FUNCTION "fc_CP_Send" : VOID
TITLE =Send CP data -PMA systembus-
//version!date    !author !change_segm!change_description
//-------+--------+-------+-----------+-------------------------------
// 1.0   !21.05.00!Kahle  ! ---       ! 1st version
// 1.1   !25.09.00!Kahle  ! 4         ! startOrder =true
//       !        !       ! 5         ! check if own station faulty
// 1.2   !10.11.00!Kahle  ! 6         ! act. tieBrk config instead of the
//       !        !       !           ! compl.config.
// 1.3   !12.03.01!Kahle  ! 6         ! if signal "OUT_uncond_semi" true the
//       !        !       !           ! signal "OUT_moreCPFaulty" is also true
// 1.4   !17.06.01!Kahle  ! 4         ! new para.: mem_actStation
//       !        !       !           ! if status =0 (Call FC5 "AG_Send")
//       !        !       !           ! --> #act_linkCond =true
//       !        !       !           ! No. of sending stations are limited per
//       !        !       !           ! call.
//       !        !       !           ! corr. delete receive buffer in case of
//       !        !       !           ! link failure
//                                                                              !
//Send CP data:
//          For each destination station exist a send data area.
//          Dependent the plant configuration are send the data to the
//          corresponding stations.
//          In case of a failure it be set an indication.
//
AUTHOR : Kahle
FAMILY : PMA71
NAME : SendFDL
VERSION : 1.4


VAR_OUTPUT
  OUT_uncond_semi : BOOL ;	//unconditional semi automatic (semi OP or semi)
  OUT_CPFaulty : BOOL ;	//At least one essential CP stations are faulty
  OUT_moreCPFaulty : BOOL ;	//more than one essential CP stations are faulty
END_VAR
VAR_IN_OUT
  mem_linkCond : DWORD ;	//link condition of each participent (=0:no order/ =1:order running)
  mem_actStation : BYTE ;	//last valid station to that data it was sent
END_VAR
VAR_TEMP
  status : WORD ;	//status value FC5 "AG_SEND"
  done : BOOL ;	//done FC5 "AG_SEND"
  error : BOOL ;	//error flag FC5 "AG_SEND"
  startOrder : BOOL ;	//=1: start order, =0:check running order
  act_linkCond : BOOL ;	//link condition of the actual participent
  no_comm : BOOL ;	//no communication possible
  send_release : BOOL ;	//send release
  newStationSend : BOOL ;	//in the loop the first order
  life_rcv : BOOL ;	//received life signal
  no_actStation : BYTE ;	//Number of stations to which data is sent
  return : INT ;	//return value function "FILL"
  REQ_ID : DWORD ;	//-- not vaild --
  data_pointer : ANY ;	//source area for the received data
  link_cnt : INT ;	//loop counter send link
  participant : DWORD ;	//CP participants (.0:G1 -.14:G15;.15:EG;.16:T1 -.19:T4;.20:S1;.21:S2
  timer_CP : INT ;	//number of the actual monitoring timer 'CP link'
  byte_bit_fail : INT ;	//byte.bit address of the CP link failure of the actual participant
  faulty_stations : DWORD ;	//faulty CP stations
  no_faulty : BYTE ;	//number of faulty CP stations
  ownStation_mask : DWORD ;	//faulty mask own station
  act_link : INT ;	//number of the actual link
  cnt_linkID : BYTE ;	//counter 'determine the link ID'
  link_fail : BOOL ;	//link failure to the actual station
END_VAR
BEGIN
NETWORK
TITLE =inital. internal variables

      CLR   ;
      =     #OUT_uncond_semi;
      =     #newStationSend;
      L     0;
      T     #no_actStation;
NETWORK
TITLE =Send CP data -inital. int.var -
// ANY-pointer: Send MPI data  (P#DB105.DBX0.0 BYTE 30)
      L     B#16#10;
      T     LB    10; //ANY-pointer: 16#10
      L     2;
      T     LB    11; //ANY-pointer: datatyp BYTE
      L     30;
      T     LW    12; //ANY-pointer: repeat factor
      L     105;
      T     LW    14; //ANY-pointer: DB No.
      L     P#DBX 0.0;
      T     LD    16; //ANY-pointer: DBX No.


NETWORK
TITLE =Check of the net configuration

      L     "prm_pma".p_tiebrkCfg;
      L     B#16#F;
      UW    ;
      L     "prm_pma".p_cfg11;
      RLD   4;
      OD    ;
      T     #participant; //actual participants

NETWORK
TITLE =Send CP data - Send data -

//verify whether the last active station is valid
      U(    ;
      L     #mem_actStation;
      L     0;
      >I    ;
      )     ;
      U(    ;
      L     20;
      L     #mem_actStation;
      >=I   ;
      )     ;
      SPB   lpsd; // if mem_actStation vaild -->jump
      L     20; // or mem_actStation not valid -->set =station 20

//Loop send data
lpsd: T     #link_cnt;
      L     #participant;
      SRD   ;
      SPZ   nxt; //participant'x' not defined ...next one

//check if destination =own station
      L     "prm_pma".p_station;
      L     #link_cnt;
      ==I   ;
      SPB   nxt; //if destination address =own station then ..next link

//actual station defined & not the own station
      L     #no_actStation;
      +     1;
      T     #no_actStation;

//source address for send data determined
      L     P#DBX 0.0;
      T     LD    16; //ANY-pointer: DBX No. -Send-
      L     #link_cnt;
      +     104;
      T     LW    14; //ANY-pointer: DB No.

//determine the link failure address
      L     #link_cnt;
      +     -1;
      L     8;
      /I    ;
      SLW   3; //convert byte ->pointer
      PUSH  ;
      RRD   16;
      OW    ;
      L     W#16#FFFF;
      UD    ;
      LAR1  ; //relative byte.bit address of the link failure of the actual participant
      T     #byte_bit_fail;

//Send data - life signal - calculate actual timer
      L     #link_cnt;
      +     100;
      T     #timer_CP; //actual Timer (participant +100)

//Send data - life signal - check the link status of each participant
      AUF   "diagn";
      UN    T [#timer_CP]; //timer stopped -->link failure
      UN    DBX [AR1,P#60.0];
      SPBN  chkT;
      S     DBX [AR1,P#60.0]; //sfc failure of the actual participant
      S     M [AR1,P#120.0]; //if monitoring time run out OR sfc failure then ...link failure
      S     #link_fail;

//link failure -reset receive buffer
      L     0;
      T     MB   255; //presetting for the receive buffer
      L     P#DBX 30.0;
      T     LD    16; //ANY-pointer: DBX No. -Receive-
      CALL "FILL" (
           BVAL                     := P#M 255.0 BYTE 1,
           RET_VAL                  := #return,
           BLK                      := #data_pointer);//the receive buffer is preset with zero

//check link status
chkT: AUF   DB [LW 14];
      U     DBX   31.7; //c_lifeG1
      L     "prm_pma".p_moniTimeMPI;
      SV    T [#timer_CP]; //..start monitoring time of the actual participant
      AUF   DB [LW 14];
      R     DBX   31.7;
      AUF   "diagn";
      R     M [AR1,P#120.0]; //reset link failure
      R     DBX [AR1,P#60.0]; //reset sfc failure of the actual participant
      R     #link_fail;

//send data -faulty order- reset commands
//      AUF   DB [LW 14]
//      L     DBD    0
//      L     DW#16#800000                //c_life
//      UD
//     T     DBD    0

//################################# especially CP Profibus ######################################################
//read the actual link condition
      L     #link_cnt;
      L     #mem_linkCond;
      SRD   ;
      SET   ;
      SPP   lnkC;
      CLR   ;
lnkC: =     #act_linkCond; //link condition of the actual participent =1 : order is finished or not started

//determine the link-ID
      L     0;
      T     #act_link;
      L     20;
lpID: T     #cnt_linkID;
      L     #participant;
      SRD   ;
      SPZ   nxID; //participant'x' not defined ...check the next ID

      L     "prm_pma".p_station;
      L     #cnt_linkID;
      ==I   ;
      SPB   nxID; //destination address =own station ...check next ID

      L     #act_link;
      +     1;
      T     #act_link;

      L     #link_cnt;
      L     #cnt_linkID;
      ==I   ;
      SPB   snd; //counter =act.link ...link ID defined
nxID: L     #cnt_linkID;
      LOOP  lpID;


//send data -check actual order running or start new order-
snd:  U     #act_linkCond;
      =     #startOrder;
//***************************************************************************************************************
      CALL "AG_SEND" (
           ACT                      := #startOrder,
           ID                       := #act_link,
           LADDR                    := "prm_pma".p_CP_add,
           SEND                     := #data_pointer,
           LEN                      := LW    12,//number of byte
           DONE                     := #done,
           ERROR                    := #error,
           STATUS                   := #status);
//***************************************************************************************************************
      L     #status; //if status =0 then ...actual order finished or no order is started
      L     0;
      ==I   ;
      =     #act_linkCond;


//################################# especially CP_Profibus ######################################################

//store the link condition
      L     #link_cnt;
      L     DW#16#80000000; //set bit32
      RLD   ; //bit position of the actual participent
      U     #act_linkCond;
      SPB   sLnk; //if act_linkCond =true then ...set
      INVD  ;
      L     #mem_linkCond;
      UW    ;
      T     #mem_linkCond; //reset link condition
      SPA   nxt;
sLnk: L     #mem_linkCond;
      OW    ;
      T     #mem_linkCond; //set link condition

//maximum numbers of station per call is achieved ?
nxt:  U(    ;
      L     #no_actStation;
      L     0;
      >I    ;
      )     ;
      U(    ;
      L     #no_actStation;
      L     DB41.DBB   40;
      >=I   ;
      )     ;
      SPB   lend; //Number of stations per call to which data are sent is achieved

//at least one defined station are verified ?
      O(    ;
      L     #no_actStation;
      L     0;
      <>I   ;
      )     ;
      O(    ;
      L     #link_cnt;
      L     1;
      <>I   ;
      )     ;
      SPB   nx;
//no defined stations are verified
      L     21;
      T     #link_cnt; //Start the verification at the beginning

//next station
nx:   L     #link_cnt;
      LOOP  lpsd;

//after the end of the loop
lend: L     #link_cnt;
      +     -1;
      T     #mem_actStation; //Storing the station which comes after the station to which data were sent at last
NETWORK
TITLE =Check if own station faulty

      L     "prm_pma".p_tiebrkCfg;
      L     B#16#F;
      UW    ;
      L     "prm_pma".p_cfg11;
      RLD   4;
      OD    ;
      T     #participant; //actual participants

      L     "prm_pma".p_station;
      L     DW#16#80000000;
      RLD   ;
      T     #ownStation_mask; // mask 'own station'

      L     #participant;
      L     #ownStation_mask;
      INVD  ;
      UD    ; //all participants without own station
      L     MD   120;
      TAD   ;
      <>D   ;
      O(    ;
      L     0;
      ==D   ;
      )     ; //if no all foreign stations faulty then ...reset own station
      SPB   Rown; //  or no faulty stations

// all stations faulty
      L     #ownStation_mask;
      TAD   ;
      L     MD   120;
      OD    ;
      T     MD   120; //set own station as faulty
      SPA   unSe;
// not all stations faulty
Rown: L     #ownStation_mask;
      INVD  ;
      TAD   ;
      L     MD   120;
      UD    ;
      T     MD   120; //set own station as o.k.

NETWORK
TITLE =Check if CP failure available
//Check if CP failure available without unessential stations
unSe: L     MD   120;
      TAD   ; //MB123,MB122,MB121,MB120
      L     DW#16#C000F;
      UD    ; //faulty tie breaker, shore connection ->dynamic uness.stations
      L     "prm_pma".p_cfgUness;
      SLD   4; //1st generator set on bit4
      OD    ;
      T     "MEM".o515_unessStation; //all uness.stations

      L     "MEM".o51_actTieCfg;
      L     B#16#F;
      UW    ;
      L     "MEM".o51_actCfg;
      RLD   4;
      OD    ; //actual participants
      L     "MEM".o515_unessStation; //all uness.stations
      INVD  ;
      UD    ; //actual paricipants without uness.stations
      L     MD   120;
      TAD   ; //MB123,MB122,MB121,MB120
      UD    ;
      T     #faulty_stations; //faulty MPI stations without unessential stations

//determine the number of faulty stations
      CALL "fc_h16NoBits" (
           IN_32bits                := #faulty_stations,
           OUT_No_bits              := #no_faulty);

      L     #no_faulty;
      L     1;
      >=I   ;
      =     #OUT_CPFaulty; //at least one ess. CP station faulty

      O(    ;
      U(    ;
      >I    ; //more than one stations faulty &release one failure
      )     ;
      U     "prm_pma".p_MPIfail_auto;
      )     ;
      O(    ;
      U(    ;
      >=I   ; //at least one ess. CP station faulty &no release one failure
      )     ;
      UN    "prm_pma".p_MPIfail_auto;
      )     ;
      =     #OUT_uncond_semi;
      =     #OUT_moreCPFaulty; //more than one CP stations faulty


END_FUNCTION




FUNCTION "fc_CP_Receive" : VOID
TITLE =Receive CP
//version!date    !author !change_segm!change_description
//-------+--------+-------+-----------+-------------------------------
// 1.0   !21.05.00!Kahle  ! ---       ! 1st version
// 1.1   !25.09.00!Kahle  ! 4         ! pointer dest. =DBX30.0
AUTHOR : Kahle
FAMILY : PMA71
NAME : Rec_FDL
VERSION : 1.1


VAR_TEMP
  return : INT ;	//return value diagnosis function
  error : BOOL ;	//error flag FC6 "AQG_RECV"
  NDR : BOOL ;	//NDR parameter FC6 "AG_RECV"
  status : WORD ;	//status paramter FC6 "AG_RECV"
  length_rcv : INT ;	//length of the received data
  station : BYTE ;	//-- not vaild --
  CP_pointer : ANY ;	//destination area for the received data
  act_link : INT ;	//number of the actual link
  link_cnt : INT ;	//loop counter send link
  participant : DWORD ;	//CP participants (.0:G1 -.14:G15;.15:EG;.16:T1 -.19:T4;.20:S1;.21:S2
END_VAR
BEGIN
NETWORK
TITLE =inital. internal variables

      L     0;
      T     #act_link;

NETWORK
TITLE =receive CP data -inital. int.var -
// ANY-pointer: received MPI data  (P#DB105.DBX30.0 BYTE 30)
      L     B#16#10;
      T     LB    10; //ANY-pointer: 16#10
      L     2;
      T     LB    11; //ANY-pointer: datatyp BYTE
      L     30;
      T     LW    12; //ANY-pointer: repeat factor
      L     105;
      T     LW    14; //ANY-pointer: DB No.
      L     P#DBX 30.0;
      T     LD    16; //ANY-pointer: DBX No.
NETWORK
TITLE =Check of the net configuration

      L     "prm_pma".p_tiebrkCfg;
      L     B#16#F;
      UW    ;
      L     "prm_pma".p_cfg11;
      RLD   4;
      OD    ;
      T     #participant; //actual participants

NETWORK
TITLE =receive MPI data
//Check if MPI data available
      L     20;
lprv: T     #link_cnt;
      L     #participant;
      SRD   ;
      SPZ   nxt; //participant'x' not defined ...next one

//check if source =own station
      L     "prm_pma".p_station;
      L     #link_cnt;
      ==I   ;
      SPB   nxt; //if destination address =own station then ..next link

//destination address for received data determined
      L     P#DBX 30.0;
      T     LD    16; //ANY-pointer: DBX No. -Send-
      L     #link_cnt;
      +     104;
      T     LW    14; //ANY-pointer: DB No.

//################################# especially CP Profibus ######################################################
//link-ID
      L     #act_link;
      +     1;
      T     #act_link;

      CALL "AG_RECV" (
           ID                       := #act_link,
           LADDR                    := "prm_pma".p_CP_add,
           RECV                     := #CP_pointer,
           NDR                      := #NDR,
           ERROR                    := #error,
           STATUS                   := #status,
           LEN                      := #length_rcv);
//################################# especially CP_Profibus ######################################################

//next station
nxt:  L     #link_cnt;
      LOOP  lprv;


END_FUNCTION

FUNCTION "fc_PMA_commCP" : VOID
TITLE =PMA internal communication
//version!date    !author !change_segm!change_description
//-------+--------+-------+-----------+-------------------------------
// 1.0   !23.05.00!Kahle  ! ---       ! 1st.valid version
// 1.1   !08.01.01!Kahle  ! 3,4       ! Ext.link failure especially TB
// 1.2   !17.06.01!Kahle  ! 2         ! new para: -mem_actStation
AUTHOR : Kahle
FAMILY : PMA71
NAME : PMAcomm
VERSION : 1.2


VAR_TEMP
  temp_forceSemi : BOOL ;
  temp_moreCPFaulty : BOOL ;
END_VAR
BEGIN
NETWORK
TITLE =CP receive
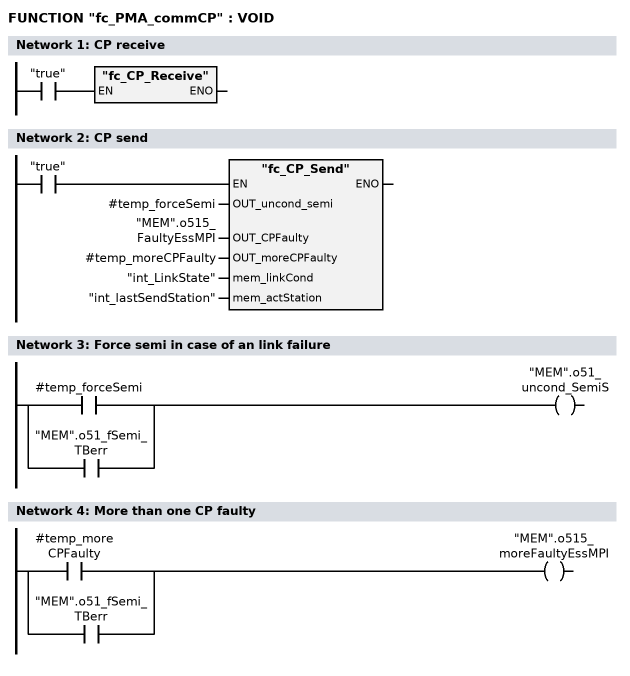
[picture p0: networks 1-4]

      U     "true";
      SPBNB _001;
      CALL "fc_CP_Receive" ;
_001: NOP   0;
NETWORK
TITLE =CP send

      U     "true";
      SPBNB _002;
      CALL "fc_CP_Send" (
           OUT_uncond_semi          := #temp_forceSemi,
           OUT_CPFaulty             := "MEM".o515_FaultyEssMPI,
           OUT_moreCPFaulty         := #temp_moreCPFaulty,
           mem_linkCond             := "int_LinkState",
           mem_actStation           := "int_lastSendStation");
_002: NOP   0;
NETWORK
TITLE =Force semi in case of an link failure

      O     #temp_forceSemi;
      O     "MEM".o51_fSemi_TBerr;
      =     "MEM".o51_uncond_SemiS;
NETWORK
TITLE =More than one CP faulty

      O     #temp_moreCPFaulty;
      O     "MEM".o51_fSemi_TBerr;
      =     "MEM".o515_moreFaultyEssMPI;
END_FUNCTION

